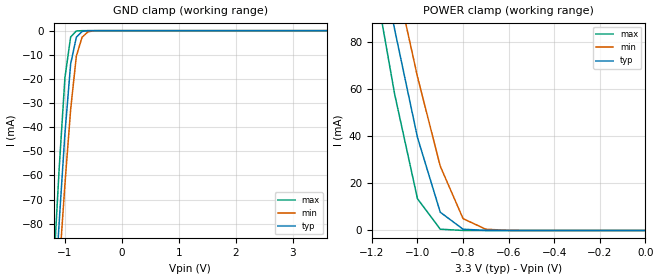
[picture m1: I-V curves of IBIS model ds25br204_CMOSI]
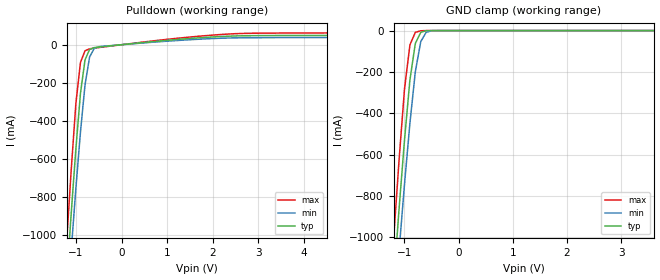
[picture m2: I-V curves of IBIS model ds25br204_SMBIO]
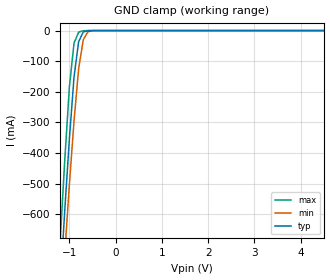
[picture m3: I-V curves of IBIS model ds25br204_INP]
|   National Semiconductor Corporation
|   IBIS Model
|   of
|   ds25br204
[IBIS Ver]   3.2
[Comment Char]   |_char
[File name]   ds25br204.ibs
[File Rev]   1.0
[Date]   11/28/2007
[Source]
[Notes]
Rev 1.0   First release.
NOTICE:   The nature of the pre-emphasis and equalization circuitry
   precludes them from being properly modeled by the simple
   I/V and V/T data in the IBIS model.  Therefore, this model
   is only valid for this device when EQ and PE pins are set
   to logic 0.
[Disclaimer]
(C) Copyright National Semiconductor Corporation 2005
   All rights reserved
   National Semiconductor Corporation hereby grants
the user of this IBIS model a non-exclusive, nontransferable
license to use this IBIS model under the following terms.
Before using this IBIS model, the user should read this
license.  If the user does not accept these terms,  the
IBIS model should be returned to National within 30 days.
   The user is granted this license only to use the
IBIS model and is not granted rights to sell, load, rent,
lease or license the IBIS model in whole or in part, or in
modified form to anyone other than user. User may modify
the IBIS model to suit its specific applications but rights
to derivative works and such modifications shall belong to
National.
   This IBIS model is provided on an "AS IS" basis and
National makes absolutely no warranty with respect to the
information contained herein.NATIONAL DISCLAIMS AND CUSTOMER
WAIVES ALL WARRANTIES, EXPRESS OR IMPLIED, INCLUDING
WARRANTIES OF MERCHANTABILITY OR FITNESS FOR A PARTICULAR
PURPOSE. The entire risk as to quality and performance is
with the Customer. ACCORDINGLY, IN NO EVENT SHALL THE
COMPANY BE LIABLE FOR ANY DAMAGES, WHETHER IN CONTRACT OR
TORT,INCLUDING ANY LOST PROFITS OR OTHER INCIDENTAL,
CONSEQUENTIAL, EXEMPLARY, OR PUNITIVE DAMAGES ARISING OUT
OF THE USE OR APPLICATION OF THE IBIS model provided in
this package.Further, National reserves the right to make
changes without notice to any product herein to improve
reliability, function, or design. National does not convey
any license under patent rights or any other intellectual
property rights, including those of third parties.
   National is not obligated to provide maintenance or support
for the licensed IBIS model.
Contact National at ATTN:INTERFACE/IBIS MODELS.
5 Foden Road, M/S 01-50, South Porltand, ME 04106
(207) 541-8467
[Copyright]
(c) Copyright 2005 National Semiconductor Corp.
[Component]   ds25br204
Si_location Pin
Timing_location Pin
[Manufacturer]   National Semiconductor Corp.
[Package]
|   TYP   MIN   MAX
R_pkg   436m   191m   537m
L_pkg   1.581n   0.879n   2.100n
C_pkg   0.119p   0.101p   0.156p
[Pin]   signal_name   model_name   R_pin   L_pin   C_pin
1   NC   NC   NA   NA   NA
2   NC   NC   NA   NA   NA
3   VDD   POWER   0.274   1.390n   0.138p
4   IN1+   ds25br204_INP   0.490   1.710n   0.116p
5   IN1-   ds25br204_INN   0.477   1.680n   0.121p
6   IN2+   ds25br204_INP   0.477   1.680n   0.122p
7   IN2-   ds25br204_INN   0.493   1.720n   0.117p
8   VDD   POWER   0.275   1.390n   0.138p
9   NC   NC   NA   NA   NA
10   NC   NC   NA   NA   NA
11   EQ2   ds25br204_CMOSI   0.515   1.850n   0.130p
12   NC   NC   NA   NA   NA
13   NC   NC   NA   NA   NA
14   SEL_in   ds25br204_CMOSI   0.364   1.210n   0.101p
15   VDD   POWER   0.191   0.879n   0.113p
16   GND   GND   0.191   0.879n   0.113p
17   NC   NC   NA   NA   NA
18   PE3   ds25br204_CMOSI   0.403   1.370n   0.103p
19   PE2   ds25br204_CMOSI   0.459   1.600n   0.107p
20   PE1   ds25br204_CMOSI   0.516   1.850n   0.130p
21   OUT3-   ds25br204_OUTN   0.572   2.100n   0.144p
22   OUT3+   ds25br204_OUTP   0.531   1.910n   0.126p
23   OUT2-   ds25br204_OUTN   0.528   1.880n   0.125p
24   OUT2+   ds25br204_OUTP   0.500   1.750n   0.116p
25   VDD   POWER   0.262   1.310n   0.138p
26   OUT1-   ds25br204_OUTN   0.480   1.670n   0.117p
27   OUT1+   ds25br204_OUTP   0.485   1.710n   0.122p
28   OUT0-   ds25br204_OUTN   0.489   1.730n   0.122p
29   OUT0+   ds25br204_OUTP   0.520   1.830n   0.117p
30   VDD   POWER   0.297   1.550n   0.156p
31   PE0   ds25br204_CMOSI   0.515   1.850n   0.125p
32   PWDN3b   ds25br204_CMOSI   0.463   1.610n   0.107p
33   PWDN2b   ds25br204_CMOSI   0.406   1.380n   0.103p
34   PWDN1b   ds25br204_CMOSI   0.364   1.220n   0.102p
35   PWDN0b   ds25br204_CMOSI   0.348   1.160n   0.103p
36   LOS2b   ds25br204_SMBIO   0.349   1.170n   0.105p
37   LOS1b   ds25br204_SMBIO   0.365   1.230n   0.104p
38   PWDNb   ds25br204_CMOSI   0.408   1.390n   0.104p
39   EQ1   ds25br204_CMOSI   0.461   1.610n   0.108p
40   NC   NC   NA   NA   NA
[Series Pin Mapping]  pin_2   model_name
4   5   input_term
6   7   input_term
[Diff Pin] inv_pin  vdiff   tdelay_typ   tdelay_min   tdelay_max
| Receiver Vth = +/-100mV
4   5   0.10   0   0   0
6   7   0.10   0   0   0
22   21   0.00   0   0   0
24   23   0.00   0   0   0
27   26   0.00   0   0   0
29   28   0.00   0   0   0
|   Model input termination resistor
[Model]   input_term
Model_type   Series
Polarity   Non-Inverting
C_comp   0.0pF   0.0pF   0.0pF
[Temperature Range] 25   85   -40
[Voltage Range]   3.3   3.0   3.6
| Resistance   ohm(typ)   ohm(min)   ohm(max)
[R Series]   100   85   115
| Models and submodels in the file (7): ds25br204_CMOSI (Input), ds25br204_SMBIO (I/O_open_sink), ds25br204_INP (Input), ds25br204_INN (Input), ds25br204_OUTP (Output), ds25br204_OUTN (Output), input_term (Series)
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[Model]   ds25br204_CMOSI
Model_type Input
Polarity Non-Inverting
Vinh=2.0
Vinl=0.8
C_comp   2pF   2pF   2pF
[Model Spec]
S_overshoot_high   3.3   3.0   3.6
S_overshoot_low   0.0   0.0   0.0
[Temperature Range]   25   85   -40
[Voltage Range]   3.3   3.0   3.6
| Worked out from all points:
|   GND clamp passes 1 mA (typ) near -0.73 V on its own axis
|   POWER clamp passes 1 mA (typ) near -0.81 V on its own axis
[GND Clamp]
-3.6V     -1.142A    -1.066A    -1.245A
-1.2V     -118.1mA   -134mA     -99.83mA
-1.1V     -79.07mA   -98.05mA   -56.77mA
-1V       -42.67mA   -63.69mA   -19.52mA
-900mV    -13.87mA   -32.72mA   -2.63mA
-800mV    -2.745mA   -10.61mA   -143.5uA
-700mV    -352.7uA   -2.771mA   -1.237uA
-600mV    -11.54uA   -555.4uA   -8.564nA
-500mV    -239.7nA   -41.77uA   -79.28pA
3.6V      33.07pA    30.43uA    28.8pA
[POWER Clamp]
-3.6V     1.477A     1.382A     1.606A
-1.2V     135.8mA    156.2mA    112.9mA
-1.1V     85.33mA    109.4mA    57.86mA
-1V       39.52mA    65.31mA    13.49mA
-900mV    7.749mA    27.31mA    544.1uA
-800mV    539.1uA    5.027mA    6.333uA
-700mV    17.37uA    520.7uA    44.05nA
-600mV    361.4nA    30.43uA    339.3pA
0V        26.4pA     28.11pA    28.8pA
[Model]   ds25br204_SMBIO
Model_type I/O_open_sink
Polarity Non-Inverting
Vinh=2.0
Vinl=0.8
C_comp   2pF   2pF   2pF
[Model Spec]
S_overshoot_high   3.3   3.0   3.6
S_overshoot_low   0.0   0.0   0.0
[Temperature Range]   25   85   -40
[Voltage Range]   3.3   3.0   3.6
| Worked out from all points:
|   slope of the pulldown table from 0 to 0.495 V, typ, clamps not added: 41.3 ohm
|   GND clamp passes 1 mA (typ) near -0.61 V on its own axis
[GND Clamp]
-3.6V     -11.36A    -10.98A    -11.96A
-1.2V     -1.218A    -1.405A    -1.004A
-1.1V     -862.1mA   -1.065A    -625.9mA
-1V       -529.7mA   -743.3mA   -283.8mA
-900mV    -238.8mA   -448.2mA   -69.16mA
-800mV    -62.25mA   -198.9mA   -8.645mA
-700mV    -8.636mA   -53.3mA    -941.4uA
-600mV    -567.5uA   -8.472mA   -96.96uA
-500mV    -43.2uA    -619.7uA   -5.593uA
3.6V      223.6pA    2.018nA    172.9pA
[Pulldown]
|V(pulldown)   I(typ)   I(min)   I(max)
-3.6V     -11.36A    -10.98A    -11.97A
-1.2V     -1.232A    -1.413A    -1.025A
-1.1V     -877.1mA   -1.074A    -648.6mA
-1V       -545.9mA   -753.6mA   -307.4mA
-900mV    -255.7mA   -459.3mA   -93.03mA
-800mV    -79.34mA   -210.4mA   -31.58mA
-700mV    -25.14mA   -65mA      -21.6mA
-600mV    -15.29mA   -19.77mA   -18.02mA
600mV     14.4mA     11.64mA    17.59mA
2.4V      45.41mA    35.58mA    56.88mA
5.8V      51.15mA    39.95mA    64.37mA
7.2V      62.06mA    49.15mA    77.21mA
[Ramp]
|   typ   min   max
dV/dt_r   1.03/200e-12   0.840/217e-12   1.238/187e-12
dV/dt_f   1.03/161e-12   0.840/194e-12   1.238/134e-12
R_load=50
|[End   ds25br204_SMBIO
[Model]   ds25br204_INP
Model_type Input
Polarity Non-Inverting
Vinh=1.25
Vinl=1.15
C_comp   1.7pF   1.7pF   1.7pF
[Model Spec]
S_overshoot_high   3.3   3.0   3.6
S_overshoot_low   0.0   0.0   0.0
[Temperature Range]   25   85   -40
[Voltage Range]   3.3   3.0   3.6
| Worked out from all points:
|   GND clamp passes 1 mA (typ) near -0.62 V on its own axis
[GND Clamp]
|V(groundclamp)   I(typ)   I(min)   I(max)
-3.6V     -7.949A    -7.688A    -8.364A
-1.2V     -837.2mA   -968.2mA   -688.4mA
-1.1V     -586.8mA   -729.1mA   -422.6mA
-1V       -353.4mA   -502.6mA   -183.7mA
-900mV    -151.8mA   -295.7mA   -40.94mA
-800mV    -36.07mA   -124.3mA   -4.991mA
-700mV    -4.641mA   -29.98mA   -506.7uA
-600mV    -299.4uA   -4.1mA     -51.64uA
-500mV    -23.36uA   -273.5uA   -3.241uA
7.2V      407.9pA    9.955nA    116.1pA
